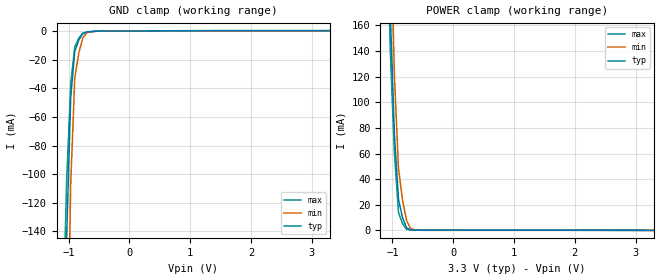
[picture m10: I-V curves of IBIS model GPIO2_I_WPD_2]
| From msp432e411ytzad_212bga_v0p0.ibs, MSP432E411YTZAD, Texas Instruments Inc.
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|   Model Cell GPIO2_I_WPD_2
[Model]   GPIO2_I_WPD_2
Model_type   Input
Polarity   Non-Inverting
Vinl =  0.8
Vinh =  2
C_comp   3.906872p   3.211855p   4.659324p
[Model Spec]
Vinl   0.8   0.8   0.8
Vinh   2   2   2
[Temperature Range]   25   125   -40
[Voltage Range]   3.3   2.97   3.63
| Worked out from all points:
|   GND clamp passes 1 mA (typ) near -0.72 V on its own axis
|   POWER clamp passes 1 mA (typ) near -0.73 V on its own axis
| Nom Voltages:
|   IBIASFET=3.3, VDDC=1.2, VDDA=3.3, VDD=3.3, GND=0, GNDA=0
| Min Voltages:
|   IBIASFET=2.97, VDDC=1.08, VDDA=2.97, VDD=2.97, GND=0, GNDA=0
| Max Voltages:
|   IBIASFET=3.63, VDDC=1.32, VDDA=3.63, VDD=3.63, GND=0, GNDA=0
[POWER_clamp]
|   voltage   I(typ)   I(min)   I(max)
-3.3V     12.79A     11.69A     13.85A
-1.1V     303.6mA    434.7mA    250.2mA
-1.033V   167.3mA    248.8mA    138.3mA
-966.7mV  74.23mA    120mA      59.57mA
-900mV    24.33mA    48.18mA    13.99mA
-833.3mV  9.892mA    23.36mA    5.308mA
-766.7mV  1.903mA    7.734mA    790uA
-700mV    360.9uA    1.315mA    440.7uA
-566.7mV  189.8uA    174.5uA    305.9uA
3.3V      -9.013pA   -34.28uA   78.8uA
[GND_clamp]
|   voltage   I(typ)   I(min)   I(max)
-3.3V     -13.29A    -11.96A    -14.49A
-1.1V     -306.4mA   -502mA     -214mA
-1.033V   -144.1mA   -263.5mA   -104.9mA
-966.7mV  -46.75mA   -107.2mA   -37.22mA
-900mV    -14.23mA   -32.82mA   -11.05mA
-833.3mV  -6.315mA   -15.27mA   -4.955mA
-766.7mV  -1.806mA   -4.706mA   -1.561mA
-700mV    -705.3uA   -1.135mA   -873.2uA
-500mV    -111.5uA   -95.34uA   -150.9uA
3.3V      162.1uA    83.88uA    277.3uA
